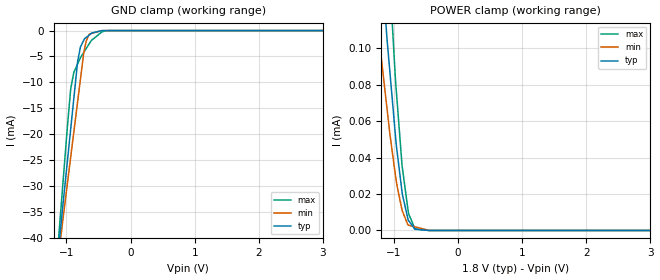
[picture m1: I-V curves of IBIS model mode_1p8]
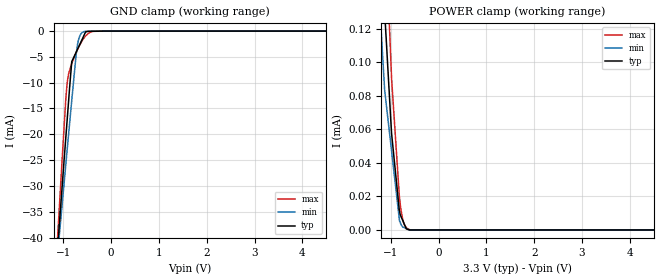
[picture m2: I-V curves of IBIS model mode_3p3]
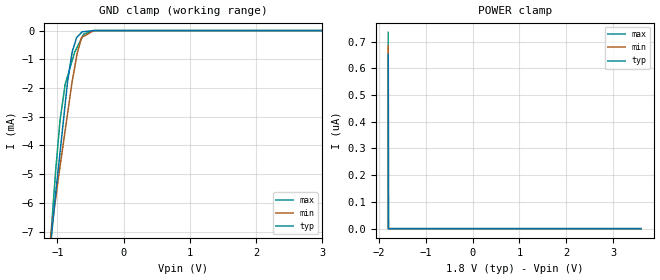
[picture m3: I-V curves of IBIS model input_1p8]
|Texas Instruments Incorporated
|90 dB SNR Low-Power Stereo Audio ADC with Microphone Bias,
|ALC, Sound Effect, Notch filter
| Marketing part#   Digital Voltage Range   Package-type   #pins
| PCM1870RHFR   1.71V - 3.6V   VQFN   24
| PCM1870RHFRG4   1.71V - 3.6V   VQFN   24
| PCM1870RHFT   1.71V - 3.6V   VQFN   24
| PCM1870RHFTG4   1.71V - 3.6V   VQFN   24
| PCM1870YZFR   1.71V - 3.6V   DSBGA   24
| PCM1870YZFT   1.71V - 3.6V   DSBGA   24
[IBIS Ver]   3.2
[File name]   pcm1870.ibs
[File Rev]   1.0
[Date]   2/17/2012
[Source]
| Texas Instruments Incorporated.
| Analog-eLab Design Center, HPA
| 12500 TI Blvd
| Dallas, TX -75243
| e-mail: elab_scm_ibis@list.ti.com
[Notes]   Revision History:
| Rev 1.0: 2/17/2012
| - Initial version of the model
| - Model generated from simulations in SPECTRE
| - Model matched to SPICE simulation
| - C_comp although listed in numerical order of value are
|   obtained from varying PVT conditions. For PVT conditions for
|   each specific value refer the buffer description under
|   respective [Model]. IBIS model user is responsible for using
|   appropriate C_comp to simulate for Signal Integrity.
| - Model names with a trailing _1p8 contains the model for
|   1.8V [1.71V and 1.89V].Model names with a trailing _3p3
|   contains the model for 3.3V [3.0V and 3.6V].
[Disclaimer]
| This model is designed as an aid for customers of Texas Instruments.
| TI and its licensors and suppliers make no warranties, either expressed
| or implied, with respect to this  model, including the warranties of
| merchantability or fitness for a particular purpose. The model is
| provided solely on an "as is" basis. The entire risk as to its quality
| and performance is with the customer.
[Copyright]
 (C) Copyright 2012 Texas Instruments Incorporated.All rights reserved.
|   PCM1870RHF
[Component]   PCM1870RHF
[Manufacturer]   TI
[Package]   |24 VQFN   -  RHF package
|   typ   min   max
R_pkg   0.06294   0.05814   0.07307
L_pkg   0.89430nH   0.81633nH   1.05968nH
C_pkg   0.091508pF   0.08460pF   0.10037pF
[Pin]  signal_name   model_name   R_pin   L_pin   C_pin
1   VCOM   TERM   0.05814   0.81633nH  0.08460pF
2   AIN2R   TERM   0.05844   0.82196nH  0.08809pF
3   AIN2L   TERM   0.06604   0.94832nH  0.09553pF
4   MODE   MODE   0.07307   1.05968nH  0.10037pF
5   MS/ADR   INPUT   0.06723   0.96269nH  0.09706pF
6   MD/SDA   IO   0.06029   0.84973nH  0.08897pF
7   MC/SCL   INPUT   0.06476   0.92410nH  0.09157pF
8   DOUT   OUTPUT   0.06401   0.91558nH  0.09319pF
9   VIO   POWER   0.02978   0.57228nH  0.11794pF
10   VDD   POWER   0.05815   0.82054nH  0.08872pF
11   DGND   GND   0.03010   0.57040nH  0.11960pF
12   SCKI   INPUT   0.06335   0.90473nH  0.09208pF
13   BCK   IO   0.06630   0.94964nH  0.09342pF
14   LRCK   IO   0.06064   0.85530nH  0.08859pF
15   TEST   GND   0.06474   0.92173nH  0.09149pF
16   AOR   TERM   0.06604   0.94832nH  0.09517pF
17   PGINR   TERM   0.05859   0.82455nH  0.08836pF
18   AOL   TERM   0.05859   0.82302nH  0.08830pF
19   PGINL   TERM   0.06604   0.94302nH  0.09452pF
20   AIN1R   TERM   0.06218   0.87846nH  0.08853pF
21   AIN1L   TERM   0.06040   0.84926nH  0.09044pF
22   MICB   TERM   0.05878   0.82277nH  0.08836pF
23   VCC   POWER   0.02909   0.55577nH  0.11323pF
24   AGND   GND   0.02960   0.55800nH  0.11611pF
1000   THERMAL_PAD   NC   0.00007   0.00128nH  0.41880pF
|   PCM1870YZF
[Component]   PCM1870YZF
[Manufacturer]   TI
[Package]   |24 DSBGA  -  YZF package
|   typ   min   max
R_pkg   0.05541   0.02966   0.07361
L_pkg   0.80718nH   0.45716nH   1.06868nH
C_pkg   0.099388pF   0.08474pF   0.14929pF
[Pin]  signal_name   model_name   R_pin   L_pin   C_pin
1   AIN1R   TERM   0.05825   0.81796nH  0.08474pF
2   AIN1L   TERM   0.05855   0.82384nH  0.08814pF
3   MICB   TERM   0.06641   0.95462nH  0.09585pF
4   VCOM   TERM   0.07361   1.06868nH  0.10096pF
5   PGINR   TERM   0.06764   0.96939nH  0.09753pF
6   PGINL   TERM   0.06048   0.85276nH  0.08912pF
7   VCC   POWER   0.06487   0.92690nH  0.09131pF
8   AGND   GND   0.06433   0.92076nH  0.09346pF
9   AOR   TERM   0.02985   0.55625nH  0.12065pF
10   AOL   TERM   0.05825   0.82219nH  0.08898pF
11   AIN2R   TERM   0.03017   0.55520nH  0.12211pF
12   AIN2L   TERM   0.06365   0.90956nH  0.09222pF
13   TEST   GND   0.00007   0.00128nH  0.03052pF
14   MODE   MODE   0.06084   0.85854nH  0.08877pF
15   MS/ADR   INPUT   0.03291   0.45716nH  0.14929pF
16   MD/SDA   IO   0.06641   0.95462nH  0.09550pF
17   LRCK   IO   0.05871   0.82654nH  0.08841pF
18   DGND   GND   0.05871   0.82495nH  0.08835pF
19   VIO   POWER   0.06641   0.94917nH  0.09485pF
20   MC/SCL   INPUT   0.06244   0.88271nH  0.08881pF
21   BCK   IO   0.06059   0.85243nH  0.09056pF
22   SCKI   INPUT   0.05891   0.82485nH  0.08845pF
23   VDD   POWER   0.02914   0.53776nH  0.11617pF
24   DOUT   OUTPUT   0.02966   0.54192nH  0.11891pF
1000   THERMAL_PAD   NC   0.00007   0.00128nH  0.41880pF
|   Model Selectors
[Model Selector] INPUT
input_1p8   1.8V digital input
input_3p3   3.3V digital input
[Model Selector] MODE
mode_1p8   1.8V digital input
mode_3p3   3.3V digital input
[Model Selector] OUTPUT
dout_1p8   1.8V digital output
dout_3p3   3.3V digital output
[Model Selector] IO
io_1p8  1.8V digital I/O
io_3p3  3.3V digital I/O
[Model Selector] TERM
term_1-8V  1.8V nominal termination
term_3-3V  3.3V nominal termination
[Model] term_1-8V
Model_type Terminator
C_comp   1.0e-20F  1.0e-20F  1.0e-20F
|   typ   min   max
[Voltage Range]   1.8V   1.71V   1.89V
[POWER Clamp Reference]   1.8V   1.71V   1.89V
[GND Clamp Reference]   0V   0V   0V
|Ambient Temperature   25   85   -40
|Junction Temperature
[Temperature Range]   26   86   -40
[Model] term_3-3V
Model_type Terminator
C_comp   1.0e-20F  1.0e-20F  1.0e-20F
|   typ   min   max
[Voltage Range]   3.3V   3.0V   3.6V
[POWER Clamp Reference]   3.3V   3.0V   3.6V
[GND Clamp Reference]   0V   0V   0V
|Ambient Temperature   25   85   -40
|Junction Temperature
[Temperature Range]   26   86   -40
| Models and submodels in the file (10): mode_1p8 (Input), mode_3p3 (Input), input_1p8 (Input), input_3p3 (Input), dout_1p8 (Output), dout_3p3 (Output), io_1p8 (I/O), io_3p3 (I/O), term_1-8V (Terminator), term_3-3V (Terminator)
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|   mode_1p8 Model
[Model]   mode_1p8
Model_type   Input
Vinl = 0.54
Vinh = 1.26
|   typ   min   max
C_comp   8.959e-13   8.859e-13   9.027e-13
[Model spec]
Vinl   0.54   0.513   0.567
Vinh   1.26   1.197   1.323
[Voltage Range]   1.8   1.71   1.89
|Ambient Temperature   25   85   -40
|Junction Temperature
[Temperature Range]   26   86   -40
[Power Clamp Reference]   1.8   1.71   1.89
[GND Clamp Reference]   0   0   0
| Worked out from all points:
|   GND clamp passes 1 mA (typ) near -0.66 V on its own axis
[GND Clamp]
|   Voltage   I(typ)   I(min)   I(max)
-1.8V     -127.5mA   -112.9mA   -149.8mA
-1.097V   -39.15mA   -40.96mA   -36.35mA
-1.051V   -33.41mA   -36.28mA   -29.18mA
-930.6mV  -18.82mA   -24.29mA   -11.14mA
-883.3mV  -13.1mA    -19.6mA    -8.07mA
-826.2mV  -6.18mA    -13.94mA   -6.489mA
-781.2mV  -3.226mA   -9.481mA   -5.245mA
-727.8mV  -1.828mA   -4.252mA   -4.197mA
-690.2mV  -1.325mA   -1.997mA   -3.463mA
-640.6mV  -840uA     -652.1uA   -2.495mA
-346.6mV  -1.437uA   0A         -18.33uA
3.6V      0A         0A         0A
[POWER Clamp]
|   Voltage   I(typ)   I(min)   I(max)
-1.8V     468.1uA    288.5uA    734.3uA
-1.334V   212.3uA    144.1uA    323.7uA
-1.203V   150.7uA    96.86uA    231.1uA
-1.133V   117.5uA    75.04uA    181.2uA
-1.105V   104.5uA    66.4uA     163.9uA
-1.063V   87.43uA    53.21uA    137.6uA
-976mV    52.32uA    30.36uA    83.91uA
-867.6mV  19.83uA    10.68uA    34.42uA
-774mV    5.342uA    2.917uA    9.87uA
-673.2mV  660.4nA    2.012uA    1.057uA
-450mV    0A         0A         0A
3.6V      0A         0A         0A
|   mode_3p3 Model
[Model]   mode_3p3
Model_type   Input
Vinl = 0.99
Vinh = 2.31
|   typ   min   max
C_comp   8.663e-13   8.474e-13   8.760e-13
[Model spec]
Vinl   0.99   0.9   1.08
Vinh   2.31   2.1   2.52
[Voltage Range]   3.3   3   3.6
|Ambient Temperature   25   85   -40
|Junction Temperature
[Temperature Range]   26   86   -40
[Power Clamp Reference]   3.3   3   3.6
[GND Clamp Reference]   0   0   0
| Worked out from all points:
|   GND clamp passes 1 mA (typ) near -0.58 V on its own axis
|   POWER clamp passes 1 mA (typ) near -2.56 V on its own axis
[GND Clamp]
|   Voltage   I(typ)   I(min)   I(max)
-3.3V     -316.9mA   -268mA     -391.9mA
-1.115V   -41.24mA   -42.61mA   -38.94mA
-1.021V   -29.54mA   -33.14mA   -24.12mA
-949.2mV  -20.65mA   -25.85mA   -13.18mA
-906mV    -15.4mA    -21.5mA    -9.078mA
-825mV    -5.93mA    -13.45mA   -6.269mA
-720mV    -3.841mA   -3.574mA   -3.911mA
-648mV    -2.41mA    -754uA     -2.54mA
-567mV    -798.7uA   -93.29uA   -1.299mA
-534.6mV  -154.3uA   -39.75uA   -941.2uA
-373.2mV  -37.44uA   -196.2nA   -41.61uA
6.6V      0A         0A         0A
[POWER Clamp]
|   Voltage   I(typ)   I(min)   I(max)
-3.3V     1.568mA    1.111mA    2.081mA
-1.944V   655.2uA    482.7uA    902.9uA
-1.185V   157.5uA    110.1uA    232.4uA
-1.131V   130.7uA    83.7uA     192.6uA
-986.7mV  57.98uA    47.45uA    91.34uA
-825mV    12.06uA    6.84uA     21.12uA
-819mV    11.18uA    5.396uA    19.21uA
-783.6mV  7.735uA    3.09uA     11.08uA
-733.2mV  4.427uA    1.545uA    4.352uA
-676.5mV  706.1nA    775.5nA    1.289uA
-624mV    156.7nA    0A         423.2nA
6.6V      0A         0A         0A
|   input_1p8 Model
[Model]   input_1p8
Model_type   Input
Vinl = 0.54
Vinh = 1.26
|   typ   min   max
C_comp   4.188e-13   4.051e-13   4.222e-13
[Model spec]
Vinl   0.54   0.513   0.567
Vinh   1.26   1.197   1.323
[Voltage Range]   1.8   1.71   1.89
|Ambient Temperature   25   85   -40
|Junction Temperature
[Temperature Range]   26   86   -40
[Power Clamp Reference]   1.8   1.71   1.89
[GND Clamp Reference]   0   0   0
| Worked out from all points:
|   GND clamp passes 1 mA (typ) near -0.79 V on its own axis
[GND Clamp]
|   Voltage   I(typ)   I(min)   I(max)
-1.8V     -24.34mA   -19.47mA   -31.1mA
-1.11V    -7.726mA   -7.352mA   -7.592mA
-1.03V    -5.786mA   -5.938mA   -5.043mA
-957.1mV  -4.216mA   -4.716mA   -3.105mA
-881.5mV  -2.58mA    -3.489mA   -1.874mA
-842.4mV  -1.748mA   -2.855mA   -1.571mA
-774mV    -735.3uA   -1.751mA   -1.04mA
-698.8mV  -218.3uA   -786.8uA   -574.9uA
-622.8mV  -41.88uA   -230.8uA   -222.4uA
-601.7mV  -36.82uA   -202.9uA   -124.7uA
-449.1mV  -344nA     -1.004uA   -1.889uA
3.6V      0A         0A         0A
[POWER Clamp]
|   Voltage   I(typ)   I(min)   I(max)
-1.8V     651.7nA    683.4nA    734.2nA
-1.797V   32.58nA    0A         69.92nA
-1.796V   0A         0A         34.96nA
-1.796V   0A         0A         0A
3.6V      0A         0A         0A
